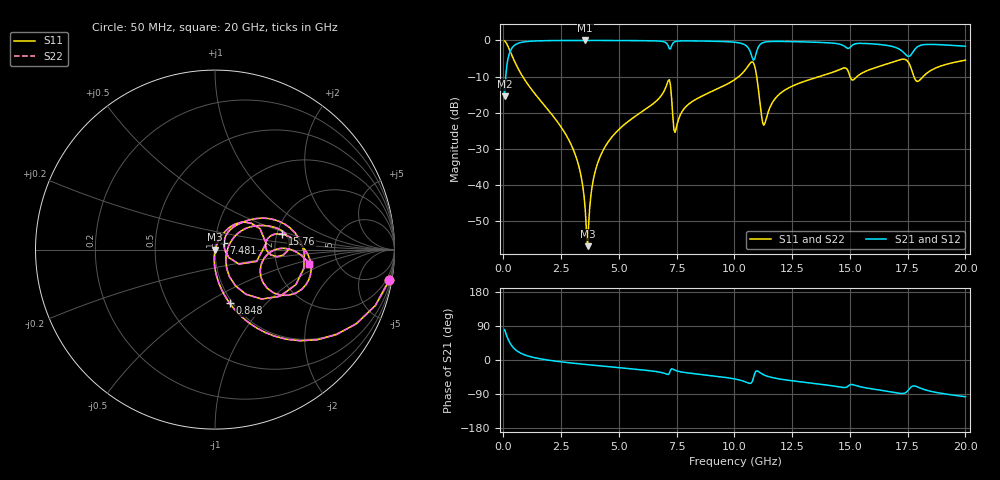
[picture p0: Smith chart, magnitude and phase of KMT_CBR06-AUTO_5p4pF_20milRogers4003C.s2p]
! Data measured by Modelithics Inc. support@modelithics.com 813-866-6335
! KEMET CBR06-AUTO 5.4pF, Pad Width= 0.851mm, Pad Length= 0.64mm, Pad Gap= 0.62mm, 20mil Rogers 4003C substrate Data, January 2022
# hz S ma R 50
! 2 Port Network Data from SP1.SP block
! freq  magS11  angS11  magS21  angS21  magS12  angS12  magS22  angS22
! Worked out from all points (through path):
!   401 points, 50 MHz to 20 GHz, reference 50 ohm
!   highest |S21| = -0.01 dB at 3.541 GHz (marker M1); lowest = -15.5 dB at 50 MHz (marker M2)
!   group delay of S21, straight-line fit = 15.2 ps
!   lowest |S11| = -56.9 dB at 3.641 GHz (marker M3), VSWR 1.00, Z = 50.1 + j0.00327 ohm
!   |S11| at or under -10 dB: 832.8 MHz to 10.19 GHz (9.356 GHz wide, 170 % of centre); 10.96 GHz to 13.68 GHz (2.717 GHz wide, 22.1 % of centre); 17.77 GHz to 18.17 GHz (401.9 MHz wide, 2.24 % of centre)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
!   |S22| runs from -56.9 to -0.1 dB; largest |S21 - S12| = 0
!   S11 on the Smith chart (normalised r, x): 50 MHz: 1, -11; 848 MHz: 0.97, -0.64; 7.481 GHz: 1.10, +0.08; 15.76 GHz: 2.14, +0.43; 20 GHz: 3.11, -0.69
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5e7  0.9856 -9.9  0.1686 80.1  0.1686 80.1  0.9856 -9.9
2.99375e8  0.696 -46.9  0.7174 43.1  0.7174 43.1  0.696 -46.9
8.48e8  0.3105 -74.6  0.9498 15.2  0.9498 15.2  0.3105 -74.6
2.74325e9  0.04717 -95.1  0.9976 -6.6  0.9976 -6.6  0.04717 -95.1
3.391625e9  0.01172 -94.3  0.9985 -10.8  0.9985 -10.8  0.01172 -94.3
3.54125e9  0.00458 -84.4  0.9985 -11.7  0.9985 -11.7  0.00458 -84.4
3.641e9  0.001422 1.3  0.9985 -12.3  0.9985 -12.3  0.001422 1.3
3.94025e9  0.014 70.0  0.9983 -14.1  0.9983 -14.1  0.014 70.0
4.389125e9  0.03328 70.6  0.9977 -16.7  0.9977 -16.7  0.03328 70.6
6.73325e9  0.1577 55.3  0.979 -31.7  0.979 -31.7  0.1577 55.3
7.13225e9  0.2766 24.9  0.8437 -38.2  0.8437 -38.2  0.2766 24.9
7.481375e9  0.06128 35.4  0.971 -28.2  0.971 -28.2  0.06128 35.4
1.0025e10  0.2886 36.8  0.9421 -50.2  0.9421 -50.2  0.2886 36.8
1.0823e10  0.4908 -23.4  0.5315 -47.6  0.5315 -47.6  0.4908 -23.4
1.127188e10  0.06706 -11.7  0.9397 -39.2  0.9397 -39.2  0.06706 -11.7
1.197012e10  0.1833 35.4  0.9688 -50.2  0.9688 -50.2  0.1833 35.4
1.336662e10  0.2944 27.2  0.9472 -61.3  0.9472 -61.3  0.2944 27.2
1.576062e10  0.3835 12.9  0.904 -74.2  0.904 -74.2  0.3835 12.9
1.670825e10  0.4837 2.5  0.8416 -83.5  0.8416 -83.5  0.4837 2.5
1.755612e10  0.4835 -31.8  0.6004 -77.6  0.6004 -77.6  0.4835 -31.8
1.795512e10  0.2718 -14.2  0.8268 -71.8  0.8268 -71.8  0.2718 -14.2
2e10  0.5324 -8.5  0.8313 -97.0  0.8313 -97.0  0.5324 -8.5
